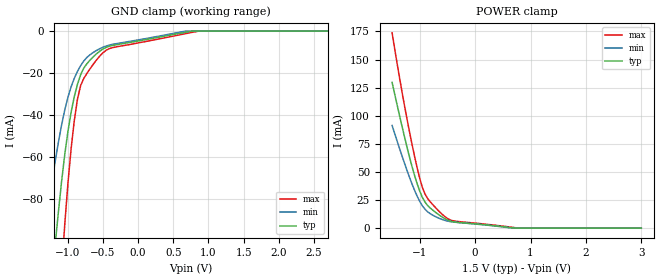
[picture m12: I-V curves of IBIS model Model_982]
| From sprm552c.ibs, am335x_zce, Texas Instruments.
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| Model based on original model for BCSHTLTCSCDDVPBFZ_SSDHV
|   Sub model DIFF_VREF_HALFTERM_5MA_10PER_1P5
[model]   Model_982
|[Description]  [1.5V-INPUT-HALFTERM:5MA-X, IND, 10%]
|   Half Thevenin termination (Rth = 100R whith RExt = 50R)
|   (ODT[1:0] = "11") VRef mode, 1.60 * RExt = 0.625 * Iout (I[2:0]
|   = "000"), 5mA nominal with Rext = 50R,Industrial temperature
|   range (-40C to 125C, 25C nominal),10% power supply tolerance
|[Input Load]   HALFTERM:5MA
|[Output Drive]
|Voltage   1.5V
|Mode   INPUT
Model_type   Input
Polarity   Non-Inverting
Vinl =  0.65
Vinh =  0.85
C_comp   1.865048p   1.676829p   1.989968p
[Model Spec]
Vinl   0.65   0.575   0.725
Vinh   0.85   0.775   0.925
[Temperature Range]   25   125   -40
[Voltage Range]   1.5   1.35   1.65
[POWER_clamp]
-1.5V     129.7mA    91.39mA    173.7mA
-1.364V   99.77mA    70.61mA    133.3mA
-1.227V   71.39mA    50.92mA    96.27mA
-1.091V   46.37mA    33.31mA    63.14mA
-1V       32.86mA    23.75mA    44.18mA
-954.5mV  27.53mA    20mA       36.48mA
-909.1mV  23.43mA    17.04mA    30.67mA
-863.6mV  20.47mA    14.8mA     26.75mA
-545.5mV  8.362mA    6.893mA    10.23mA
-363.6mV  5.436mA    5.279mA    6.251mA
772.7mV   0A         0A         96.76uA
3V        0A         0A         0A
[GND_clamp]
-1.5V     -225.1mA   -136.2mA   -370.9mA
-1.318V   -152.8mA   -92.39mA   -252.4mA
-1.182V   -102.2mA   -62.27mA   -167.2mA
-1.136V   -86.57mA   -53.23mA   -140.5mA
-1.045V   -59.05mA   -37.71mA   -92.52mA
-954.5mV  -38.74mA   -26.58mA   -56.21mA
-863.6mV  -25.32mA   -19.19mA   -32.42mA
-772.7mV  -17.57mA   -14.19mA   -22.5mA
-636.4mV  -12.2mA    -10.12mA   -15.67mA
-409.1mV  -7.21mA    -6.658mA   -8.348mA
863.6mV   0A         0A         0A
3V        0A         0A         0A
